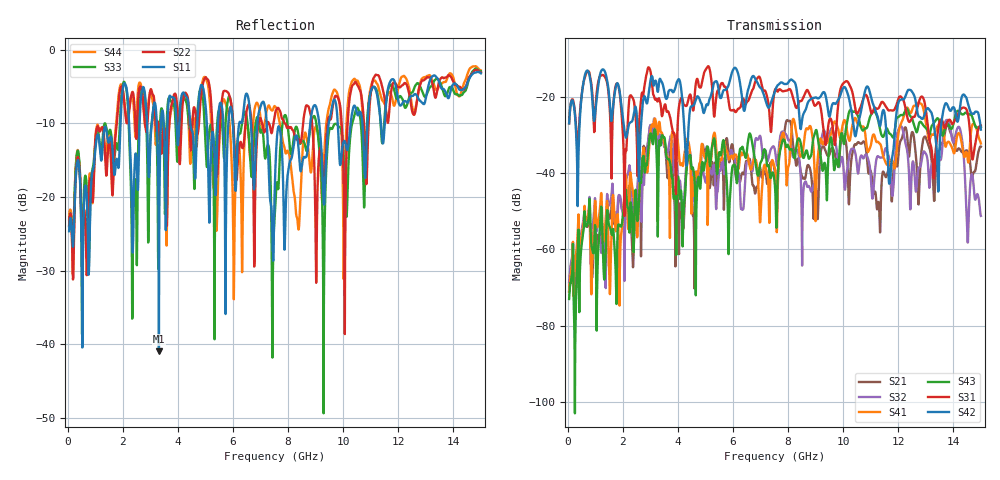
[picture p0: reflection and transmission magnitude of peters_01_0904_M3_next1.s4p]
# MHZ S RI R 50.00
! FREQ  S11  S12  S13  S14
!  S21  S22  S23  S24
!  S31  S32  S33  S34
!  S41  S42  S43  S44
!  REAL  IMAG  REAL  IMAG  REAL  IMAG  REAL  IMAG
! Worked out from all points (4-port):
!   1496 points, 50 MHz to 15 GHz, reference 50 ohm
!   strongest paths, dB at 50 MHz, 3.79 GHz, 7.53 GHz, 11.27 GHz, 15 GHz:
!     S42: -27.0, -18.5, -18.4, -25.8, -28.6
!     S31: -27.0, -28.2, -18.1, -23.1, -27.5
!     S43: -73.0, -41.3, -44.1, -26.2, -27.9
!     S41: -71.2, -29.4, -39.1, -31.8, -32.3
!     S32: -68.6, -31.8, -34.3, -35.6, -51.3
!     S21: -70.9, -36.6, -40.7, -47.7, -33.1
!   lowest |S11| = -40.9 dB at 3.31 GHz (marker M1), VSWR 1.02, Z = 50.9 + j0.158 ohm
!   |S11| at or under -10 dB: start of sweep to 1.916 GHz; 7.225 GHz to 8.805 GHz (1.58 GHz wide, 19.7 % of centre); 9.803 GHz to 10.27 GHz (468.4 MHz wide, 4.67 % of centre)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
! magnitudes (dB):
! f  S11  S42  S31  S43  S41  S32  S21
! 50 MHz  -24.6  -27.0  -27.0  -73.0  -71.2  -68.6  -70.9
! 3.31 GHz  -40.9  -16.4  -20.4  -33.8  -26.8  -31.4  -32.0
! 4.58 GHz  -13.5  -22.2  -22.6  -39.9  -46.0  -43.7  -53.4
! 8.01 GHz  -16.3  -16.2  -18.2  -33.0  -38.3  -31.4  -26.4
! 11.29 GHz  -7.5  -26.5  -23.0  -26.8  -32.0  -35.7  -47.8
! 13.78 GHz  -6.4  -22.1  -26.6  -27.2  -32.0  -26.1  -27.3
! 15 GHz  -3.2  -28.6  -27.5  -27.9  -32.3  -51.3  -33.1
